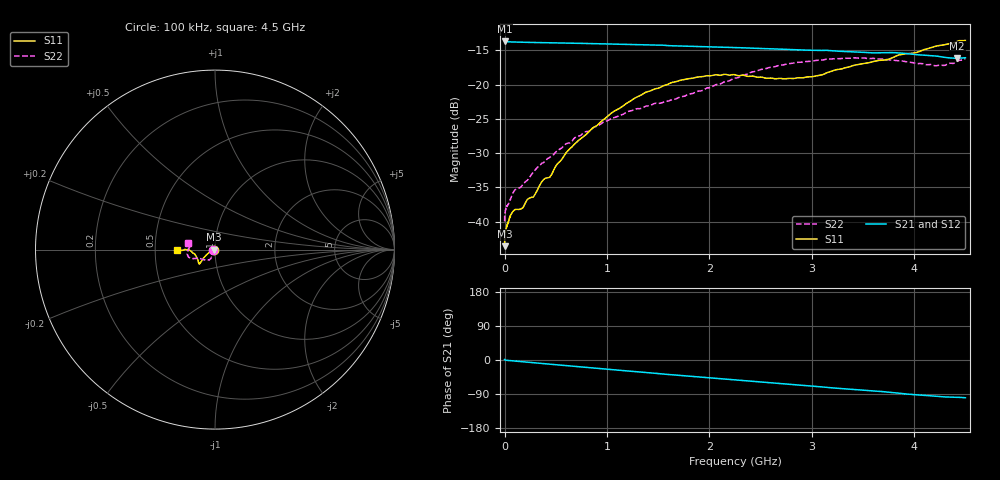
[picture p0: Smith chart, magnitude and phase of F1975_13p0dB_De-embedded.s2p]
! Integrated Device Technology
! Corporate Headquarters
! 6024 Silver Creek Valley Road
! San Jose, CA 95138  USA
! Phone:  1-408-284-8200
! Toll Free:  1-800-223-1366
! Webpage:  http://www.idt.com/
! Timing and RF Division
! 515 Groton Road, Suite 102
! Westford, MA 01886-6024
! Device:  F1975
! Description: 6-bit, 75 ohm, 0.5 dB Digital Step Attenuator
! Frequency:  5.0 MHz -  3.00 GHz
! Package:  4x4 mm QFN Plastic Package: 20 pin
! Ports:  2 RF, 11 DC
!  Pin  1  = D5 (16 dB)
!  Pin  2  = RF1  =  Port 1
!  Pin  3  = Serial Data In (DATA)
!  Pin  4  = Serial Clock (CLK)
!  Pin  5  = Serial Latch Enable (LE)
!  Pin  6  = VDD
!  Pin  7  = NC
!  Pin  8  = NC
!  Pin  9  = NC
!  Pin 10  = GND
!  Pin 11  = GND
!  Pin 12  = NC
!  Pin 13  = VMODE
!  Pin 14  = RF2  =  Port 2
!  Pin 15  = D4 (8 dB)
!  Pin 16  = D3 (4 dB)
!  Pin 17  = D2 (2 dB)
!  Pin 18  = NC
!  Pin 19  = D1 (1 dB)
!  Pin 20  = D0 (0.5 dB)
! State:  26
! Atten State:  13.0 dB
! Voltage:  +3.30 Volts
! Current:  0.592 mA
! Data:  The device was measured on a F1975 evaluation board which has
!  individual transmission lines to the RF pins.  Data was collected
!  using a calibrated network analyzer.  The evaluation board was
!  de-embedded using Automatic Fixture Removal (AFR).
!  The reference plane is the edge of the package pin.
! Misc:
!  Action Tracker AT0415
! Date Measured:  2018-02-08
! Date:  2018-03-26  MJV
! Note:
!  Integrated Device Technology supplies this data as a sample of measured
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# GHz S dB R 75
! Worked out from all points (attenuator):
!   291 points, 100 kHz to 4.5 GHz, reference 75 ohm
!   highest |S21| = -13.65 dB at 100 kHz (marker M1); lowest = -16.2 dB at 4.42 GHz (marker M2)
!   lowest |S11| = -43.6 dB at 100 kHz (marker M3), VSWR 1.01, Z = 74 - j0.0137 ohm
!   |S11| at or under -10 dB: start of sweep to end of sweep
!   |S22| runs from -40.0 to -16.1 dB; largest |S21 - S12| = 0.00013
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0.0001  -43.59 -179.2  -13.65 1.2  -13.65 1.2  -39.96 -177.7
0.0005  -42.75 -176.0  -13.67 1.1  -13.67 1.1  -39.50 -177.3
0.002  -42.01 -174.9  -13.70 0.8  -13.69 0.8  -38.95 -175.3
0.011  -41.17 -172.5  -13.73 -0.5  -13.72 -0.5  -38.16 -171.5
0.08  -38.54 -164.3  -13.78 -2.3  -13.78 -2.3  -35.85 -157.1
0.18  -37.96 -160.9  -13.82 -4.8  -13.82 -4.8  -34.54 -136.8
0.22  -36.80 -160.9  -13.83 -5.7  -13.83 -5.7  -34.00 -131.7
0.28  -36.42 -158.6  -13.85 -7.2  -13.85 -7.2  -32.77 -128.7
0.38  -33.88 -157.7  -13.88 -9.6  -13.88 -9.6  -31.38 -120.0
0.44  -33.53 -156.6  -13.89 -11.0  -13.89 -11.0  -30.64 -116.5
0.6  -29.96 -156.1  -13.94 -14.8  -13.94 -14.8  -28.64 -114.7
0.76  -27.73 -151.0  -13.98 -18.6  -13.98 -18.6  -27.18 -114.3
1.06  -23.98 -146.2  -14.08 -25.7  -14.08 -25.7  -24.86 -115.6
1.52  -20.41 -140.1  -14.24 -36.2  -14.24 -36.2  -22.72 -127.1
1.88  -18.91 -137.4  -14.44 -44.4  -14.43 -44.4  -21.00 -142.3
2.26  -18.61 -139.8  -14.60 -52.8  -14.59 -52.8  -19.03 -153.9
2.68  -19.09 -153.3  -14.82 -62.1  -14.81 -62.1  -17.19 -158.5
3.02  -18.80 -166.7  -14.99 -69.3  -14.99 -69.3  -16.53 -162.5
3.76  -16.24 -179.6  -15.33 -85.0  -15.32 -85.0  -16.38 -177.2
4.2  -14.44 -178.5  -15.82 -95.4  -15.81 -95.4  -17.24 170.9
4.42  -13.68 -177.8  -16.16 -98.5  -16.15 -98.4  -16.59 167.6
4.5  -13.55 -179.6  -16.08 -99.7  -16.07 -99.6  -16.17 166.5
